(* Logix 5000 AddOnInstructionDefinition export YAI_Assy_170_101_EIP_Hz; software revision 21.03 *)

ADD_ON_INSTRUCTION YAI_Assy_170_101_EIP_Hz   (* revision 1.0, vendor Yaskawa America, Inc. *)
// YAI Assembly 170 and 101
// Help:
// This add-on instruction is for use with input assemblie 170 and output assembly 101.
// Node_Input_Assy is defined as the node's input assembly integer array.
// Node_Output_Assy is defined as the node's output assembly integer array.
// Torque limit/reference, torque compensation and torque output variables are only available with A1000.
VAR_IN_OUT
   Node_Input_Assy : AB:ETHERNET_MODULE_INT_24Bytes:I:0; {required}   // Input assembly words
   Node_Output_Assy : AB:ETHERNET_MODULE_INT_8Bytes:O:0; {required}   // Output assembly words
END_VAR
VAR_INPUT
   RunFwd : BOOL; {visible}   // Forward run command
   RunRev : BOOL; {visible}   // Reverse run command
   MFI_3 : BOOL; {visible}   // Multi-function input 3
   MFI_4 : BOOL; {visible}   // Multi-function input 4
   MFI_5 : BOOL; {visible}   // Multi-function input 5
   MFI_6 : BOOL; {visible}   // Multi-function input 6
   MFI_7 : BOOL; {visible}   // Multi-function input 7
   MFI_8 : BOOL; {visible}   // Multi-function input 8
   External_Fault : BOOL;   // External fault command (EF0)
   FaultReset : BOOL; {visible}   // Fault reset command
   MFO_1 : BOOL; {visible}   // Multi-function output (M1-M2 for A/P1000, MA/MB/MC for V1000)
   MFO_2 : BOOL; {visible}   // Multi-function output (M3-M4 for A/P1000, P1 for V1000)
   MFO_3 : BOOL; {visible}   // Multi-function output (M5-M6 for A/P1000, P2 for V1000)
   Freq_Ref : REAL; {visible}   // Frequency reference command in Hz (xx.xx resolution)
   Torq_Ref_Limit : REAL; {visible}   // Torque reference/limit (A1000 only)
   Torq_Comp : REAL; {visible}   // Torque compensation command (A1000 only)
END_VAR
VAR_OUTPUT
   Running : BOOL; {access Read Only, visible}   // Drive running forward status bit
   ZSP : BOOL; {access Read Only, visible}   // Drive zero speed status bit
   RunningRev : BOOL; {access Read Only, visible}   // Drive running reverse status bit
   Reset : BOOL; {access Read Only, visible}   // Drive reset command status bit
   At_Speed : BOOL; {access Read Only, visible}   // Drive at commanded speed status bit
   Ready : BOOL; {access Read Only, visible}   // Drive ready status bit
   Alarm : BOOL; {access Read Only, visible}   // Drive alarm status bit
   Faulted : BOOL; {access Read Only, visible}   // Drive faulted status bit
   OPE : BOOL; {access Read Only}   // OPE alarm/fault present
   UV : BOOL; {access Read Only}   // Drive in UV (undervoltage) state status bit
   NetCtrlStatus : BOOL; {access Read Only, visible}   // Drive network run source status bit (1 = source coming from network)
   MFO_1_Status : BOOL; {access Read Only, visible}   // Drive multi-function output 1 (M1-M2 for A/P1000, MA/MB/MC for V1000) status
   MFO_2_Status : BOOL; {access Read Only, visible}   // Drive multi-function output 1 (M3-M4 for A/P1000, P1 for V1000) status
   MFO_3_Status : BOOL; {access Read Only, visible}   // Drive multi-function output 1 (M5-M6 for A/P1000, P2 for V1000) status
   ZSV : BOOL; {access Read Only, visible}   // Drive zero servo completed status bit
   Motor_Speed : REAL; {access Read Only, visible}   // Motor speed in Hz (xx.xx resolution)
   Custom_In_1 : INT; {access Read Only}
   Custom_In_2 : INT; {access Read Only}
   Custom_In_3 : INT; {access Read Only}
   Custom_In_4 : INT; {access Read Only}
   Custom_In_5 : INT; {access Read Only}
   Custom_In_6 : INT; {access Read Only}
   Custom_In_7 : INT; {access Read Only}
   Custom_In_8 : INT; {access Read Only}
   Custom_In_9 : INT; {access Read Only}
   Custom_In_10 : INT; {access Read Only}
END_VAR
VAR
   FRef_Convert : DINT;
   FOut_Convert : REAL;
   FOut_Temp : REAL;
   TRef_Convert : INT;
   TComp_Convert : INT;
   TOut_Convert : REAL;
   TOut_Temp : REAL;
   IOut_Temp : REAL;
   IOut_Convert : REAL;
   AO1_Convert : INT;
   AO2_Convert : INT;
   Motor_Speed_Temp : REAL;
   Motor_Speed_Convert : REAL;
   Freq_Cmd_Temp : REAL;
   Freq_Cmd_Convert : REAL;
   AI1_Temp : REAL;
   AI1_Convert : REAL;
   AI2_Temp : REAL; {access None}
   AI2_Convert : REAL; {access None}
   AI3_Temp : REAL; {access None}
   AI3_Convert : REAL; {access None}
END_VAR

ROUTINE Logic   (* ladder *)
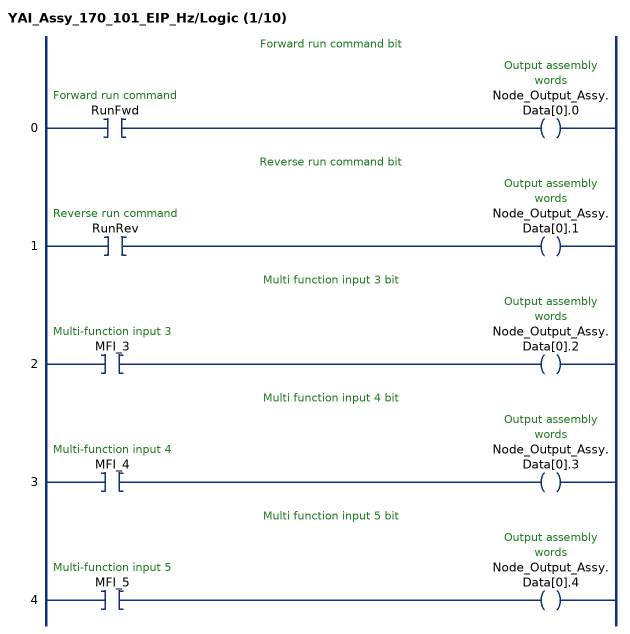
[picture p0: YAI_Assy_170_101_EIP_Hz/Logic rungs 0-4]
   // Forward run command bit
   0: XIC(RunFwd)OTE(Node_Output_Assy.Data[0].0);
   // Reverse run command bit
   1: XIC(RunRev)OTE(Node_Output_Assy.Data[0].1);
   // Multi function input 3 bit
   2: XIC(MFI_3)OTE(Node_Output_Assy.Data[0].2);
   // Multi function input 4 bit
   3: XIC(MFI_4)OTE(Node_Output_Assy.Data[0].3);
   // Multi function input 5 bit
   4: XIC(MFI_5)OTE(Node_Output_Assy.Data[0].4);
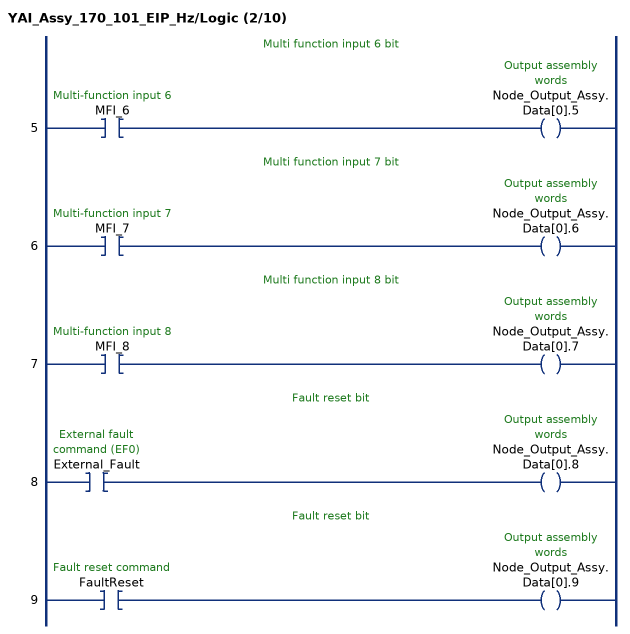
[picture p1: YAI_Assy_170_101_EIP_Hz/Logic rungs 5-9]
   // Multi function input 6 bit
   5: XIC(MFI_6)OTE(Node_Output_Assy.Data[0].5);
   // Multi function input 7 bit
   6: XIC(MFI_7)OTE(Node_Output_Assy.Data[0].6);
   // Multi function input 8 bit
   7: XIC(MFI_8)OTE(Node_Output_Assy.Data[0].7);
   // Fault reset bit
   8: XIC(External_Fault)OTE(Node_Output_Assy.Data[0].8);
   // Fault reset bit
   9: XIC(FaultReset)OTE(Node_Output_Assy.Data[0].9);
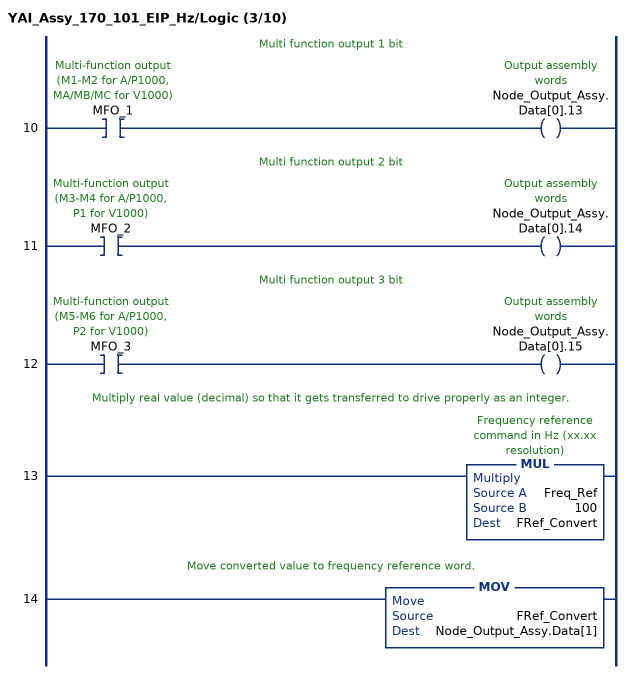
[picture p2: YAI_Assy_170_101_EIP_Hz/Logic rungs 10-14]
   // Multi function output 1 bit
   10: XIC(MFO_1)OTE(Node_Output_Assy.Data[0].13);
   // Multi function output 2 bit
   11: XIC(MFO_2)OTE(Node_Output_Assy.Data[0].14);
   // Multi function output 3 bit
   12: XIC(MFO_3)OTE(Node_Output_Assy.Data[0].15);
   // Multiply real value (decimal) so that it gets transferred to drive properly as an integer.
   13: MUL(Freq_Ref,100,FRef_Convert);
   // Move converted value to frequency reference word.
   14: MOV(FRef_Convert,Node_Output_Assy.Data[1]);
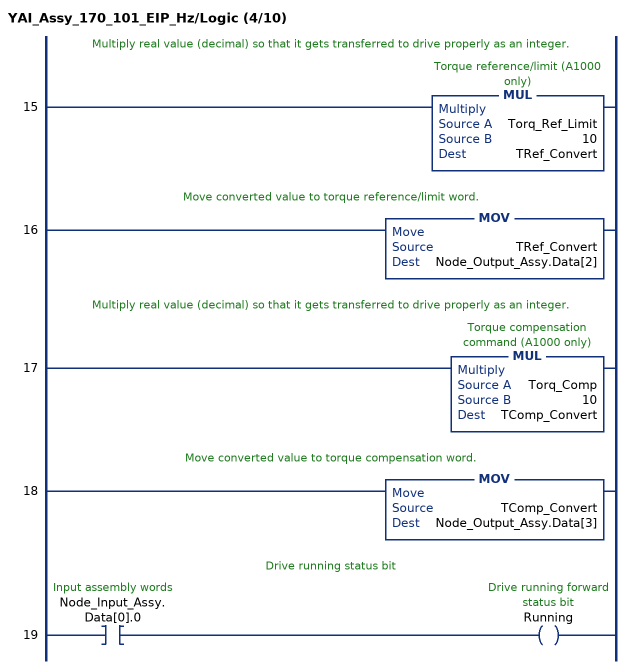
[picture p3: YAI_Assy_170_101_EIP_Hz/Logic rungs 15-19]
   // Multiply real value (decimal) so that it gets transferred to drive properly as an integer.
   15: MUL(Torq_Ref_Limit,10,TRef_Convert);
   // Move converted value to torque reference/limit word.
   16: MOV(TRef_Convert,Node_Output_Assy.Data[2]);
   // Multiply real value (decimal) so that it gets transferred to drive properly as an integer.
   17: MUL(Torq_Comp,10,TComp_Convert);
   // Move converted value to torque compensation word.
   18: MOV(TComp_Convert,Node_Output_Assy.Data[3]);
   // Drive running status bit
   19: XIC(Node_Input_Assy.Data[0].0)OTE(Running);
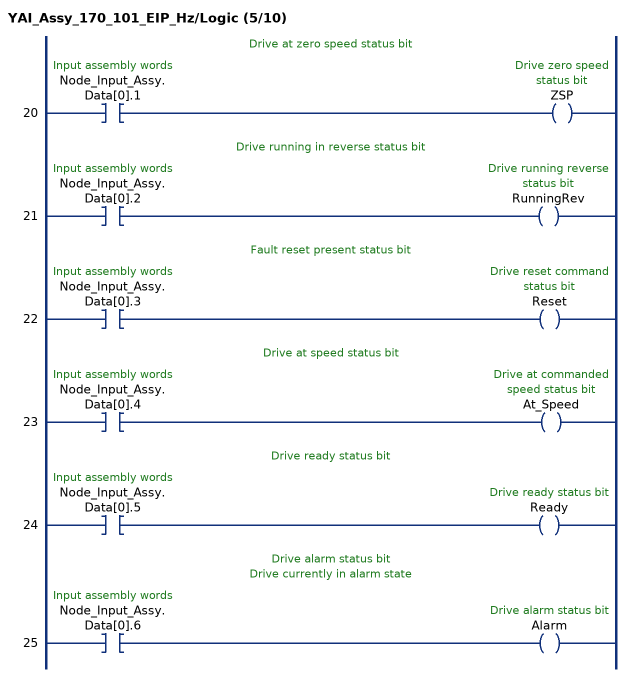
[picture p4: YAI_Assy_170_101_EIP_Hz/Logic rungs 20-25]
   // Drive at zero speed status bit
   20: XIC(Node_Input_Assy.Data[0].1)OTE(ZSP);
   // Drive running in reverse status bit
   21: XIC(Node_Input_Assy.Data[0].2)OTE(RunningRev);
   // Fault reset present status bit
   22: XIC(Node_Input_Assy.Data[0].3)OTE(Reset);
   // Drive at speed status bit
   23: XIC(Node_Input_Assy.Data[0].4)OTE(At_Speed);
   // Drive ready status bit
   24: XIC(Node_Input_Assy.Data[0].5)OTE(Ready);
   // Drive alarm status bit
   // Drive currently in alarm state
   25: XIC(Node_Input_Assy.Data[0].6)OTE(Alarm);
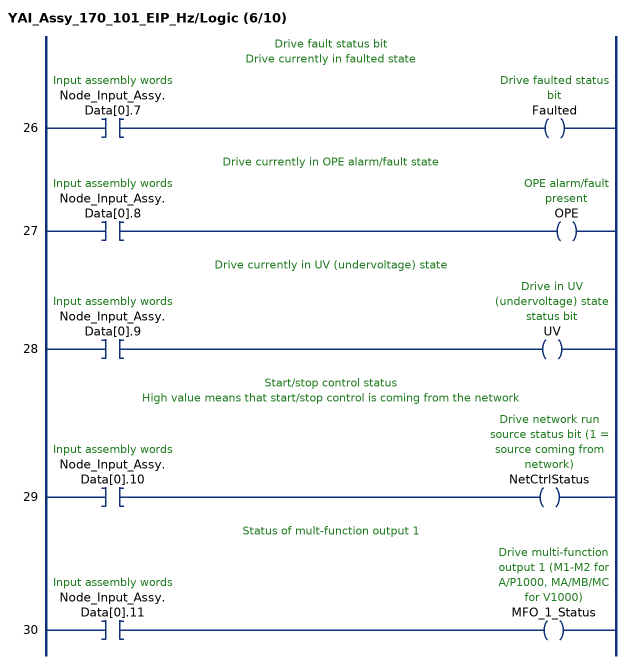
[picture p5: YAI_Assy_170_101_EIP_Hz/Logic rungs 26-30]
   // Drive fault status bit
   // Drive currently in faulted state
   26: XIC(Node_Input_Assy.Data[0].7)OTE(Faulted);
   // Drive currently in OPE alarm/fault state
   27: XIC(Node_Input_Assy.Data[0].8)OTE(OPE);
   // Drive currently in UV (undervoltage) state
   28: XIC(Node_Input_Assy.Data[0].9)OTE(UV);
   // Start/stop control status
   // High value means that start/stop control is coming from the network
   29: XIC(Node_Input_Assy.Data[0].10)OTE(NetCtrlStatus);
   // Status of mult-function output 1
   30: XIC(Node_Input_Assy.Data[0].11)OTE(MFO_1_Status);
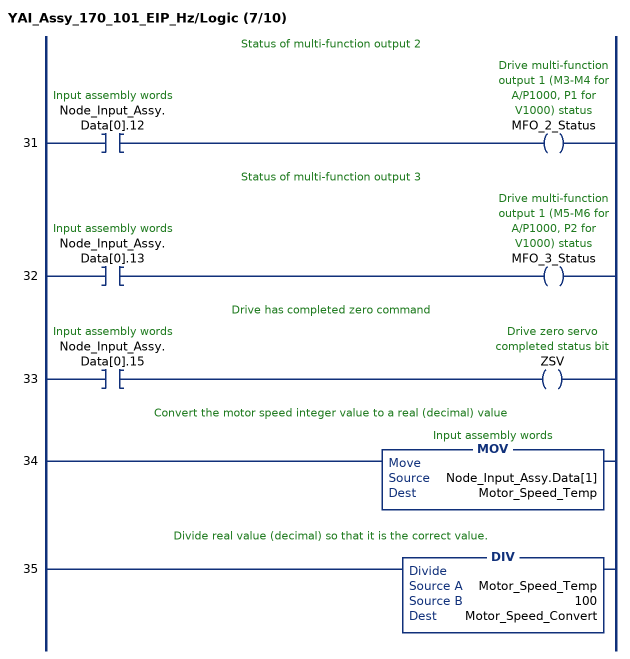
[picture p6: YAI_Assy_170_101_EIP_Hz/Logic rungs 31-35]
   // Status of multi-function output 2
   31: XIC(Node_Input_Assy.Data[0].12)OTE(MFO_2_Status);
   // Status of multi-function output 3
   32: XIC(Node_Input_Assy.Data[0].13)OTE(MFO_3_Status);
   // Drive has completed zero command
   33: XIC(Node_Input_Assy.Data[0].15)OTE(ZSV);
   // Convert the motor speed integer value to a real (decimal) value
   34: MOV(Node_Input_Assy.Data[1],Motor_Speed_Temp);
   // Divide real value (decimal) so that it is the correct value.
   35: DIV(Motor_Speed_Temp,100,Motor_Speed_Convert);
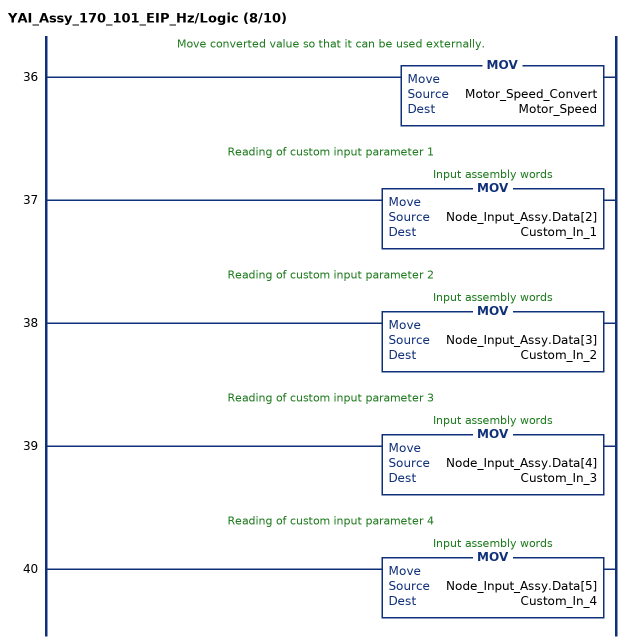
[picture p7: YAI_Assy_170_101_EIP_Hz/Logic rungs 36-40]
   // Move converted value so that it can be used externally.
   36: MOV(Motor_Speed_Convert,Motor_Speed);
   // Reading of custom input parameter 1
   37: MOV(Node_Input_Assy.Data[2],Custom_In_1);
   // Reading of custom input parameter 2
   38: MOV(Node_Input_Assy.Data[3],Custom_In_2);
   // Reading of custom input parameter 3
   39: MOV(Node_Input_Assy.Data[4],Custom_In_3);
   // Reading of custom input parameter 4
   40: MOV(Node_Input_Assy.Data[5],Custom_In_4);
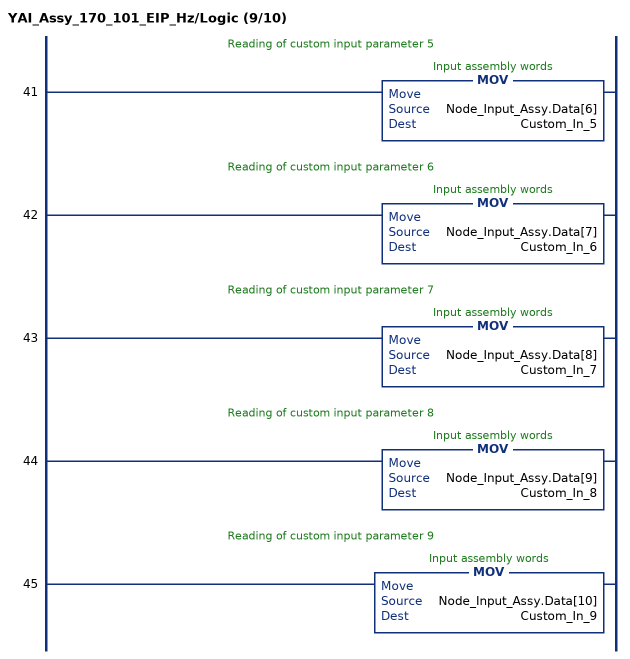
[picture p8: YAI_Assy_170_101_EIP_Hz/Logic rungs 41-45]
   // Reading of custom input parameter 5
   41: MOV(Node_Input_Assy.Data[6],Custom_In_5);
   // Reading of custom input parameter 6
   42: MOV(Node_Input_Assy.Data[7],Custom_In_6);
   // Reading of custom input parameter 7
   43: MOV(Node_Input_Assy.Data[8],Custom_In_7);
   // Reading of custom input parameter 8
   44: MOV(Node_Input_Assy.Data[9],Custom_In_8);
   // Reading of custom input parameter 9
   45: MOV(Node_Input_Assy.Data[10],Custom_In_9);
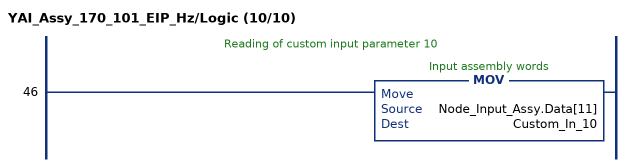
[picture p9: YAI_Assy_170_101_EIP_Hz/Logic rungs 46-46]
   // Reading of custom input parameter 10
   46: MOV(Node_Input_Assy.Data[11],Custom_In_10);
END_ROUTINE
END_ADD_ON_INSTRUCTION
